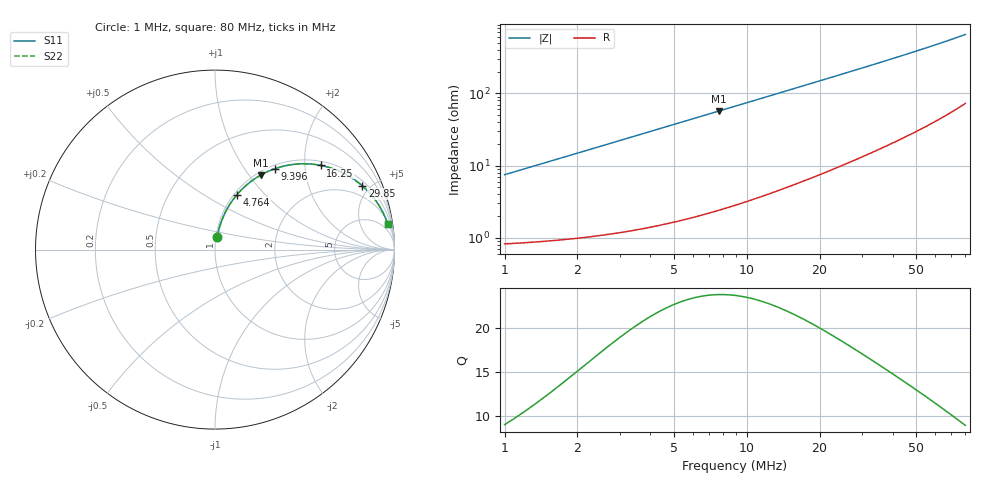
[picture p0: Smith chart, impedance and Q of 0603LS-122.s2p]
# MHz S MA R 50
!Freq  MagS11  AngS11  MagS21  AngS21  MagS12  AngS12  MagS22  AngS22
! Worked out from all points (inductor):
!   801 points, 1 MHz to 80 MHz, reference 50 ohm
!   read as one part in series: L = 1.18 uH near 1.022 MHz
!   highest Q = 23.8 at 7.672 MHz (marker M1), where L = 1.18 uH
!   S11 on the Smith chart (normalised r, x): 1 MHz: 1.02, +0.15; 4.764 MHz: 1.03, +0.71; 9.396 MHz: 1.06, +1.39; 16.25 MHz: 1.11, +2.42; 29.85 MHz: 1.26, +4.48; 80 MHz: 2, +13
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1  0.07377 79.5  0.9892 -4.2  0.9892 -4.2  0.07377 79.5
1.300725  0.09553 79.4  0.9869 -5.5  0.9869 -5.5  0.09553 79.4
1.619347  0.1184 78.9  0.984 -6.8  0.984 -6.8  0.1184 78.9
1.994053  0.1451 77.9  0.9799 -8.3  0.9799 -8.3  0.1451 77.9
2.42871  0.1757 76.5  0.9742 -10.1  0.9742 -10.1  0.1757 76.5
2.925884  0.2099 74.8  0.9666 -12.1  0.9666 -12.1  0.2099 74.8
3.467383  0.2463 72.9  0.9571 -14.2  0.9571 -14.2  0.2463 72.9
4.764044  0.3287 68.3  0.9299 -19.2  0.9299 -19.2  0.3287 68.3
6.095715  0.4056 63.6  0.8969 -23.9  0.8969 -23.9  0.4056 63.6
7.672499  0.4861 58.5  0.8537 -29.1  0.8537 -29.1  0.4861 58.5
9.396254  0.5611 53.5  0.8043 -34.1  0.8043 -34.1  0.5611 53.5
11.57048  0.6382 47.9  0.7426 -39.6  0.7426 -39.6  0.6382 47.9
14.16999  0.7094 42.3  0.6734 -45.1  0.6734 -45.1  0.7094 42.3
16.24954  0.7535 38.5  0.6231 -48.8  0.6231 -48.8  0.7535 38.5
18.73663  0.7948 34.7  0.5693 -52.5  0.5693 -52.5  0.7948 34.7
21.369  0.8284 31.2  0.5194 -55.8  0.5194 -55.8  0.8284 31.2
27.34217  0.8795 25.4  0.4291 -61.4  0.4291 -61.4  0.8795 25.4
29.84659  0.8941 23.5  0.3987 -63.2  0.3987 -63.2  0.8941 23.5
40.56122  0.9328 17.6  0.3025 -68.5  0.3025 -68.5  0.9328 17.6
53.9277  0.9554 13.2  0.2284 -72.2  0.2284 -72.2  0.9554 13.2
67.13769  0.9666 10.4  0.1808 -74.2  0.1808 -74.2  0.9666 10.4
80  0.9727 8.5  0.148 -75.2  0.148 -75.2  0.9727 8.5
